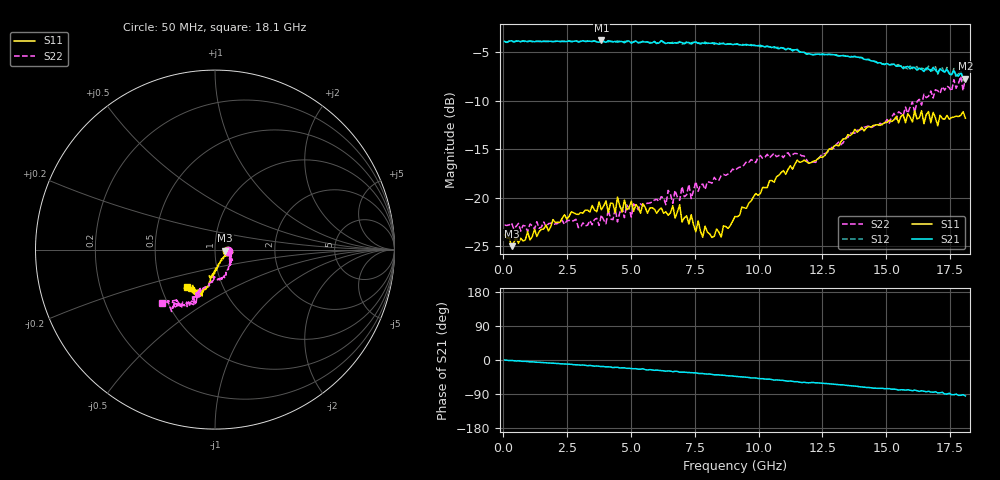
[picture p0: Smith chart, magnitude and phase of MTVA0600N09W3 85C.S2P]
! Network Analyzer HP8720D.06.14 Serial No. US36140669
! 10 May 2005  15:13:03
! Frequency  S11  S21  S12  S22
# HZ  S  DB R 50
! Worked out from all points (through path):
!   201 points, 50 MHz to 18.1 GHz, reference 50 ohm
!   highest |S21| = -3.83 dB at 3.841 GHz (marker M1); lowest = -7.7 dB at 18.1 GHz (marker M2)
!   group delay of S21, straight-line fit = 14.4 ps
!   lowest |S11| = -25.0 dB at 320.8 MHz (marker M3), VSWR 1.12, Z = 55.9 - j0.59 ohm
!   |S11| at or under -10 dB: start of sweep to end of sweep
!   |S22| runs from -23.5 to -7.5 dB; largest |S21 - S12| = 0.027
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5e7  -23.80 -5.2  -3.92 -0.0  -3.96 -0.4  -22.80 -4.0
3.2075e8  -24.97 -5.3  -3.85 -1.1  -3.90 -1.3  -22.59 -5.8
3.1185e9  -21.57 -11.9  -3.85 -13.2  -3.89 -13.7  -22.57 -18.0
3.8405e9  -21.23 -6.2  -3.83 -17.3  -3.89 -17.1  -21.77 -22.2
4.382e9  -21.55 -9.1  -3.92 -19.3  -4.00 -19.9  -21.14 -17.5
4.47225e9  -19.92 -9.9  -3.99 -19.2  -3.87 -20.3  -22.48 -15.2
4.65275e9  -21.48 -12.0  -3.93 -20.7  -4.00 -21.6  -21.04 -14.6
4.743e9  -20.23 -6.9  -4.07 -20.7  -3.93 -21.3  -22.05 -18.7
6.09675e9  -21.24 -8.8  -4.09 -27.3  -4.02 -28.0  -20.37 -22.8
6.7285e9  -22.07 -3.9  -4.05 -29.8  -4.12 -29.8  -19.23 -32.7
6.909e9  -20.72 -8.6  -4.01 -32.2  -3.94 -32.3  -20.26 -33.9
6.99925e9  -22.49 -10.2  -4.05 -32.2  -4.20 -32.4  -18.84 -31.7
7.36025e9  -21.74 -18.5  -4.20 -33.4  -4.07 -34.5  -20.07 -32.4
7.8115e9  -24.05 -28.1  -4.08 -35.6  -4.12 -36.4  -18.58 -39.8
8.5335e9  -24.04 -55.0  -4.14 -40.0  -4.16 -40.6  -17.72 -54.4
9.075e9  -21.92 -69.7  -4.22 -43.1  -4.21 -43.7  -17.18 -61.3
1.060925e10  -18.40 -91.7  -4.47 -53.0  -4.59 -52.9  -15.42 -76.7
1.21435e10  -16.25 -99.3  -5.30 -59.4  -5.27 -60.2  -16.31 -90.6
1.512175e10  -12.01 -107.4  -6.33 -75.6  -6.34 -76.7  -12.33 -109.1
1.79195e10  -11.52 -129.3  -7.13 -93.0  -6.89 -90.9  -7.51 -125.1
1.800975e10  -11.15 -128.2  -7.65 -91.8  -7.97 -94.7  -9.00 -127.5
1.81e10  -11.81 -126.8  -7.74 -94.8  -7.41 -96.4  -7.57 -134.8
